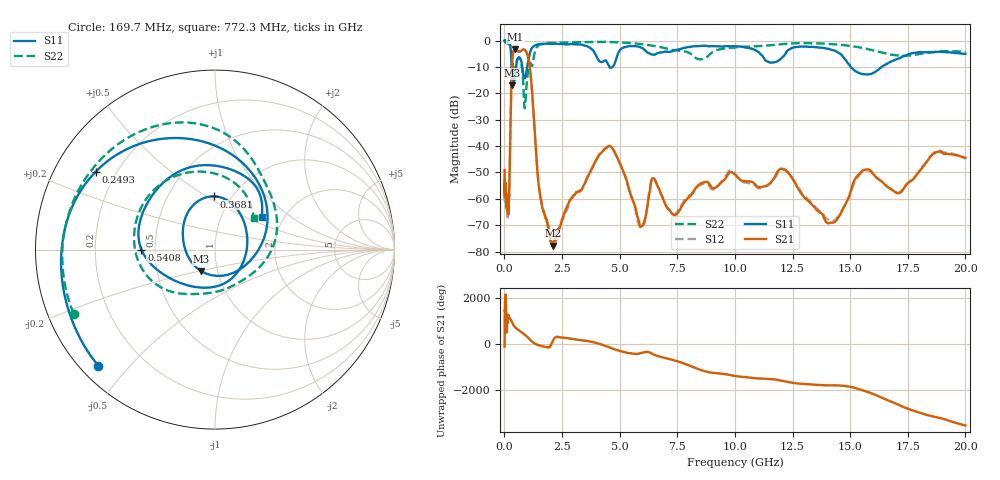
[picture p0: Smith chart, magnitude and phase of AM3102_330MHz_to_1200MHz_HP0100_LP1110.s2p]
! Date/Time: Tue, Sep 11, 2018 5:13 PM
! Network Analyzer: Agilent Technologies E8362B Rev: A.07.50.63
! Sweep from 0.010 to 20.000 GHz, 1601 Points, Sweep Type: LOG
! Power Supply: 4.949 V, 0.001 A
# Hz S DB R 50
!freq MagS11 AngS11 MagS21 AngS21 MagS12 AngS12 MagS22 AngS22
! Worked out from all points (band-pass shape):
!   1601 points, 10 MHz to 20 GHz, reference 50 ohm
!   highest |S21| = -3.30 dB at 478 MHz (marker M1); lowest = -77.7 dB at 2.094 GHz (marker M2)
!   |S21| within 3 dB of the highest: 353.7 MHz to 1.03 GHz (676.1 MHz wide, 97.7 % of centre)
!   lowest |S11| = -16.9 dB at 330 MHz (marker M3), VSWR 1.33, Z = 41.8 - j10.2 ohm
!   |S11| at or under -10 dB: 307.8 MHz to 508.4 MHz (200.6 MHz wide, 49.1 % of centre); 772.9 MHz to 988.2 MHz (215.3 MHz wide, 24.5 % of centre); 15.03 GHz to 16.37 GHz (1.345 GHz wide, 8.57 % of centre)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
!   |S22| runs from -25.7 to -0.3 dB; largest |S21 - S12| = 0.012
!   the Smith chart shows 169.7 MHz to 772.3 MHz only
!   S11 on the Smith chart (normalised r, x): 169.7 MHz: 0.05, -0.41; 249.3 MHz: 0.12, +0.29; 368.1 MHz: 0.83, +0.54; 540.8 MHz: 0.42, -0.00; 772.3 MHz: 1.55, +0.63
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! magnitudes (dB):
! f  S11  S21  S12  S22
! 10 MHz  0.0  -49.0  -55.3  -0.3
! 35.55 MHz  0.0  -58.2  -61.3  -0.6
! 126.4 MHz  -0.4  -61.5  -62.4  -1.1
! 169.7 MHz  -0.7  -64.5  -62.6  -1.3
! 199.4 MHz  -1.1  -58.6  -61.5  -1.4
! 249.3 MHz  -2.0  -39.5  -39.6  -1.8
! 330 MHz  -16.9  -8.8  -8.8  -5.8
! 368.1 MHz  -10.6  -5.5  -5.6  -8.6
! 447.2 MHz  -14.4  -3.4  -3.5  -12.7
! 478 MHz  -12.7  -3.3  -3.3  -11.6
! 540.8 MHz  -7.7  -3.8  -3.8  -7.9
! 772.3 MHz  -10.0  -3.6  -3.6  -11.1
! 882.2 MHz  -14.3  -3.6  -3.6  -25.7
! 1.103 GHz  -4.9  -10.1  -10.0  -8.5
! 1.59 GHz  -1.4  -60.5  -60.3  -1.3
! 2.094 GHz  -1.2  -77.7  -77.9  -0.8
! 4.457 GHz  -8.3  -40.4  -40.3  -0.5
! 5.652 GHz  -2.1  -62.4  -62.5  -1.1
! 12.09 GHz  -6.1  -48.6  -48.8  -1.3
! 14.14 GHz  -3.4  -69.0  -68.3  -1.3
! 15.62 GHz  -12.7  -49.0  -49.3  -3.0
! 20 GHz  -5.0  -44.4  -44.7  -4.2
